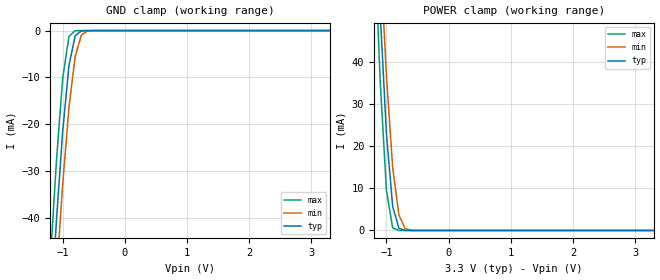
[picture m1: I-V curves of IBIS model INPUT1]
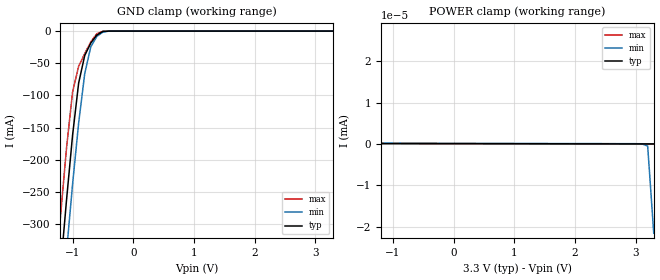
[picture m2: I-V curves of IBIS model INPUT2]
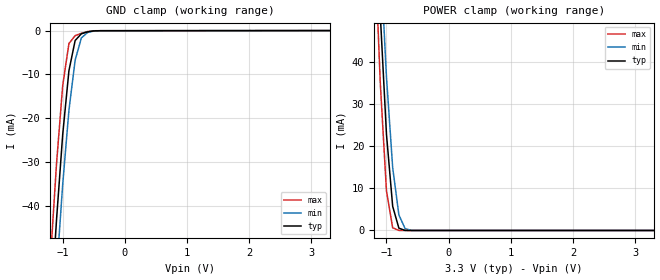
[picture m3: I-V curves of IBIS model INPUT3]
|   DIODES INCORPORATED
|   IBIS Model of PI6CG33802C
|   Product Family: 6CG
|   TQFN (ZL-48) Package
[IBIS Ver] 4.0
[Comment char] |_char
[File Name] pi6cg33802c_zl_reva.ibs
[File Rev] 1.0
[Source] File originated at Diodes Incorporated.
[Date] 04/02/2020
[Disclaimer] (C) Copyright DIODES INCORPORATED
   All rights reserved
  Diodes Incorporated hereby grants the user of
  this IBIS model a non-exclusive, nontransferable license to
  use this IBIS model under the following terms.
  This IBIS model is provided on an "AS IS" basis and Diodes
  makes absolutely no warranty with respect to the information
  contained herein. DIODES DISCLAIMS AND CUSTOMER WAIVES ALL
  WARRANTIES, EXPRESSED OR IMPLIED, INCLUDING WARRANTIES OF
  MERCHANTABILITY OR FITNESS FOR A PARTICULAR PURPOSE. The
  entire risk as to quality and performance is with the customer.
  Accordingly, in no event shall the company be liable for any
  damages, whether in contract or tort, including any lost
  profits or other incidental, consequential, exemplary, or
  punitive damages arising out of the use or application of the
  IBIS model provided in this package. Further, Diodes reserves
  the right to make changes without notice to any product herein
  to improve reliability, function, or design. Diodes does not
  convey any license under patent rights or any other intellectual
  property rights, including those of third parties.
  The user is granted this license only to use the IBIS model
  and is not granted rights to sell, load, rent, lease or license
  the IBIS model in whole or in part, or in modified form to anyone
  other than user. User may modify the IBIS model to suit its specific
  application but rights to derivative works and such modifications
  shall belong to Diodes.
  Diodes is not obligated to provide maintenance or support
  for the licensed IBIS model.
  Contact Diodes at ATTN: APPLICATION ENGINEERING / IBIS MODELS
  1545 Barber Ln. Milpitas, CA 95035
[Component] PI6CG33802C
[Manufacturer] Diodes Incorporated.
[Package]
| Variable   typ   min   max
R_pkg   0.03902ohm   0.02922ohm   0.04882ohm
L_pkg   0.79998nH   0.76828nH   0.83168nH
C_pkg   0.19606pF   0.17176pF   0.22036pF
[Pin]  signal_name   model_name   R_pin   L_pin   C_pin
1   SS_SEL_TRI   INPUT5   0.04882   0.83168nH   0.22036pF
2   GND_XTAL   GND   0.04490   0.81900nH   0.21064pF
3   XTAL_IN/CLK   INPUT1   0.04098   0.80632nH   0.20092pF
4   XTAL_OUT   OUTPUT   0.03706   0.79364nH   0.19120pF
5   VDD_OSC   POWER   0.03314   0.78096nH   0.18148pF
6   VDD_REFOUT   POWER   0.02922   0.76828nH   0.17176pF
7   SADR/REFOUT   IO   0.02922   0.76828nH   0.17176pF
8   GND_REFOUT   GND   0.03314   0.78096nH   0.18148pF
9   GND_DIG   GND   0.03706   0.79364nH   0.19120pF
10   SCLK   INPUT2   0.04098   0.80632nH   0.20092pF
11   SDATA   IO_OS   0.04490   0.81900nH   0.21064pF
12   VDD_DIG   POWER   0.04882   0.83168nH   0.22036pF
13   VDDO   POWER   0.04882   0.83168nH   0.22036pF
14   OE0#   INPUT3   0.04490   0.81900nH   0.21064pF
15   Q0+   HCSL_OUT   0.04098   0.80632nH   0.20092pF
16   Q0-   HCSL_OUT   0.03706   0.79364nH   0.19120pF
17   OE1#   INPUT3   0.03314   0.78096nH   0.18148pF
18   Q1+   HCSL_OUT   0.02922   0.76828nH   0.17176pF
19   Q1-   HCSL_OUT   0.02922   0.76828nH   0.17176pF
20   VDD   POWER   0.03314   0.78096nH   0.18148pF
21   VDDO   POWER   0.03706   0.79364nH   0.19120pF
22   GND   GND   0.04098   0.80632nH   0.20092pF
23   Q2+   HCSL_OUT   0.04490   0.81900nH   0.21064pF
24   Q2-   HCSL_OUT   0.04882   0.83168nH   0.22036pF
25   OE2#   INPUT3   0.04882   0.83168nH   0.22036pF
26   Q3+   HCSL_OUT   0.04490   0.81900nH   0.21064pF
27   Q3-   HCSL_OUT   0.04098   0.80632nH   0.20092pF
28   OE3#   INPUT3   0.03706   0.79364nH   0.19120pF
29   GNDA   GND   0.03314   0.78096nH   0.18148pF
30   VDDA   POWER   0.02922   0.76828nH   0.17176pF
31   VDDO   POWER   0.02922   0.76828nH   0.17176pF
32   Q4+   HCSL_OUT   0.03314   0.78096nH   0.18148pF
33   Q4-   HCSL_OUT   0.03706   0.79364nH   0.19120pF
34   OE4#   INPUT3   0.04098   0.80632nH   0.20092pF
35   Q5+   HCSL_OUT   0.04490   0.81900nH   0.21064pF
36   Q5-   HCSL_OUT   0.04882   0.83168nH   0.22036pF
37   OE5#   INPUT3   0.04882   0.83168nH   0.22036pF
38   VDD   POWER   0.04490   0.81900nH   0.21064pF
39   VDDO   POWER   0.04098   0.80632nH   0.20092pF
40   GND   GND   0.03706   0.79364nH   0.19120pF
41   Q6+   HCSL_OUT   0.03314   0.78096nH   0.18148pF
42   Q6-   HCSL_OUT   0.02922   0.76828nH   0.17176pF
43   OE6#   INPUT3   0.02922   0.76828nH   0.17176pF
44   Q7+   HCSL_OUT   0.03314   0.78096nH   0.18148pF
45   Q7-   HCSL_OUT   0.03706   0.79364nH   0.19120pF
46   OE7#   INPUT3   0.04098   0.80632nH   0.20092pF
47   VDDO   POWER   0.04490   0.81900nH   0.21064pF
48   PD#   INPUT4   0.04882   0.83168nH   0.22036pF
| Models and submodels in the file (9): INPUT1 (Input), INPUT2 (Input), INPUT3 (Input), INPUT4 (Input), INPUT5 (Input), OUTPUT (Output), IO (I/O), IO_OS (I/O_open_sink), HCSL_OUT (Output)
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[Model] INPUT1
Model_type Input
Vinl = 825mV
Vinh = 2.75V
| variable   typ   min   max
C_comp   4.138pF   4.098pF   4.182pF
[Voltage Range]   3.3V   3.135V   3.465V
[GND Clamp Reference]   0.000V   0.000V   0.000V
[POWER Clamp Reference]   3.3V   3.135V   3.465V
[temperature range]   25   85   -40
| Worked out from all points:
|   GND clamp passes 1 mA (typ) near -0.79 V on its own axis
|   POWER clamp passes 1 mA (typ) near -0.81 V on its own axis
[GND Clamp]
| Voltage   I(typ)   I(min)   I(max)
-3.3V     -611mA     -617mA     -607mA
-1.2V     -62.2mA    -74.3mA    -49.3mA
-1.1V     -40.5mA    -52.6mA    -27.7mA
-1V       -21.5mA    -32.9mA    -10.2mA
-900mV    -7.54mA    -16.5mA    -1.27mA
-800mV    -1.13mA    -5.57mA    -24.2uA
-700mV    -53.2uA    -958uA     -202nA
-600mV    -1.35uA    -74.3uA    -1.53nA
3.3V      9.9pA      35.5pA     9.41pA
[POWER Clamp]   |Note: Vtable = Vcc - Voutput
| Voltage   I(typ)   I(min)   I(max)
-3.3V     1.02A      977mA      1.08A
-1.2V     86.3mA     99mA       71.7mA
-1.1V     51.3mA     65.5mA     35.1mA
-1V       22.8mA     36.4mA     9.39mA
-900mV    5.72mA     14.9mA     638uA
-800mV    544uA      3.68mA     8.25uA
-700mV    18.7uA     441uA      62.5nA
-600mV    428nA      26.6uA     460pA
3.3V      -9.9pA     -97pA      -9.41pA
[Model] INPUT2
Model_type Input
Vinl = 825mV
Vinh = 2.75V
| variable   typ   min   max
C_comp   2.377pF   2.375pF   2.379pF
[Voltage Range]   3.3V   3.135V   3.465V
[GND Clamp Reference]   0.000V   0.000V   0.000V
[POWER Clamp Reference]   3.3V   3.135V   3.465V
[temperature range]   25   85   -40
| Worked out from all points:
|   GND clamp passes 1 mA (typ) near -0.51 V on its own axis
|   POWER clamp passes 1 mA (typ) near -2.41 V on its own axis
[GND Clamp]
| Voltage   I(typ)   I(min)   I(max)
-3.3V     -3.1A      -3.15A     -3.08A
-1.3V     -486mA     -569mA     -402mA
-1.2V     -372mA     -455mA     -289mA
-1.1V     -263mA     -344mA     -182mA
-1V       -162mA     -238mA     -94.7mA
-900mV    -80.8mA    -143mA     -54.6mA
-800mV    -38mA      -66.3mA    -35.1mA
-700mV    -18.5mA    -24.4mA    -16.7mA
-600mV    -6.12mA    -8.27mA    -3.99mA
-500mV    -639uA     -1.47mA    -152uA
-400mV    -17.1uA    -85.9uA    -1.09uA
3.3V      65.7pA     151pA      64.9pA
[POWER Clamp]   |Note: Vtable = Vcc - Voutput
| Voltage   I(typ)   I(min)   I(max)
-3.3V     678mA      594mA      765mA
-2.2V     101nA      80.9nA     101nA
-2.1V     2.3nA      3.56nA     863pA
-2V       153pA      374pA      113pA
3.1V      4.4pA      39pA       7.18pA
3.2V      2.41pA     -514pA     5.21pA
3.3V      0A         -21.6nA    3.25pA
[Model] INPUT3
Model_type Input
Vinl = 825mV
Vinh = 2.75V
| variable   typ   min   max
C_comp   0.482pF   0.477pF   0.488pF
[Voltage Range]   3.3V   3.135V   3.465V
[GND Clamp Reference]   0.000V   0.000V   0.000V
[POWER Clamp Reference]   3.3V   3.135V   3.465V
[temperature range]   25   85   -40
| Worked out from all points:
|   GND clamp passes 1 mA (typ) near -0.72 V on its own axis
|   POWER clamp passes 1 mA (typ) near -0.81 V on its own axis
[GND Clamp]
| Voltage   I(typ)   I(min)   I(max)
-3.3V     -806mA     -784mA     -851mA
-1.2V     -65.6mA    -77.9mA    -52.7mA
-1.1V     -43.3mA    -55.5mA    -30.5mA
-1V       -23.7mA    -35.1mA    -12.5mA
-900mV    -9.15mA    -18.2mA    -2.93mA
-800mV    -2.24mA    -6.72mA    -1.13mA
-700mV    -702uA     -1.66mA    -594uA
-600mV    -266uA     -406uA     -185uA
-500mV    -41.5uA    -86.4uA    -13.4uA
3.3V      27.3uA     28.7uA     25.2uA
[POWER Clamp]   |Note: Vtable = Vcc - Voutput
| Voltage   I(typ)   I(min)   I(max)
-3.3V     1.02A      977mA      1.08A
-1.2V     86.3mA     99mA       71.7mA
-1.1V     51.3mA     65.5mA     35.1mA
-1V       22.8mA     36.4mA     9.39mA
-900mV    5.72mA     14.9mA     638uA
-800mV    544uA      3.68mA     8.25uA
-700mV    18.7uA     441uA      62.5nA
-600mV    428nA      26.6uA     460pA
3.3V      -9.9pA     -97pA      -9.41pA
